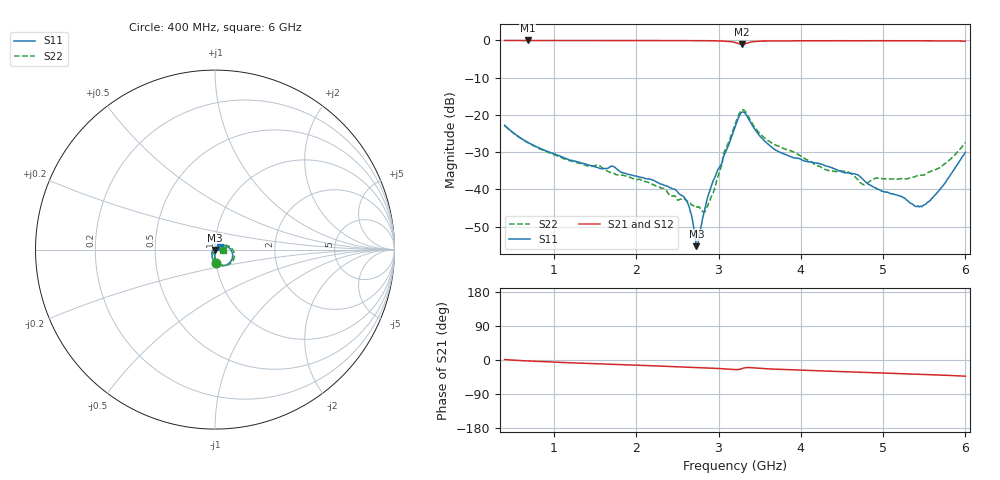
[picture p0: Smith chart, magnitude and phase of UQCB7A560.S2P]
!  Part Number  UQCB7A560	Mounting Orientation: Vertical
!  Description: RF capacitors
!  Application: Coupling, Bypass, Tuning, DC Block
!  Filters, Matching
# GHZ S DB R 50
! Freq  |S11|  S11 Ph  |S21|  S21 Ph  |S12|  S12 Ph  |S22|  S22 Ph
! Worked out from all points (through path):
!   801 points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, 400 MHz to 6 GHz, reference 50 ohm
!   highest |S21| = -0.03 dB at 680 MHz (marker M1); lowest = -1.1 dB at 3.284 GHz (marker M2)
!   group delay of S21, straight-line fit = 20 ps
!   lowest |S11| = -55.2 dB at 2.731 GHz (marker M3), VSWR 1.00, Z = 50.1 - j0.16 ohm
!   |S11| at or under -10 dB: start of sweep to end of sweep
!   |S22| runs from -46.0 to -18.6 dB; largest |S21 - S12| = 0.0013
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0.4  -22.79 -87.7  -0.04 1.2  -0.04 1.2  -22.83 -87.2
0.68  -27.32 -90.5  -0.03 -2.5  -0.03 -2.5  -27.43 -89.2
1.338  -32.94 -96.5  -0.04 -8.5  -0.04 -8.5  -33.13 -89.2
1.716  -33.77 -100.4  -0.06 -11.5  -0.05 -11.5  -35.56 -90.7
2.269  -38.22 -105.6  -0.06 -15.8  -0.06 -15.8  -39.29 -82.3
2.598  -42.64 -105.4  -0.09 -18.4  -0.09 -18.4  -42.83 -58.9
2.654  -45.63 -108.2  -0.08 -18.9  -0.08 -18.9  -43.63 -51.8
2.731  -55.20 -66.7  -0.09 -19.6  -0.08 -19.6  -44.64 -36.9
2.759  -52.81 -23.0  -0.09 -19.8  -0.09 -19.8  -44.62 -31.1
2.815  -46.87 9.1  -0.09 -20.4  -0.09 -20.4  -45.98 -12.1
2.864  -42.31 19.7  -0.10 -20.9  -0.10 -20.9  -44.49 13.6
3.2  -23.28 15.1  -0.56 -25.3  -0.56 -25.3  -22.55 16.4
3.284  -19.27 -29.9  -1.09 -22.8  -1.09 -22.8  -18.68 -24.5
3.515  -25.99 -106.6  -0.20 -22.3  -0.20 -22.3  -25.29 -89.3
3.676  -29.21 -119.2  -0.15 -24.2  -0.15 -24.2  -27.87 -96.9
4.138  -32.67 -135.7  -0.12 -28.0  -0.12 -28.0  -32.76 -111.4
4.579  -35.53 -151.1  -0.10 -31.4  -0.11 -31.4  -35.38 -98.2
4.761  -37.40 -165.3  -0.12 -32.6  -0.12 -32.6  -38.70 -85.5
5.069  -40.88 -167.3  -0.10 -35.0  -0.10 -35.0  -37.16 -63.5
5.496  -44.14 104.7  -0.13 -38.2  -0.13 -38.2  -36.17 -30.2
5.706  -39.55 60.4  -0.14 -39.8  -0.13 -39.9  -33.89 -11.9
6  -30.02 25.3  -0.23 -42.7  -0.23 -42.7  -27.40 0.2
